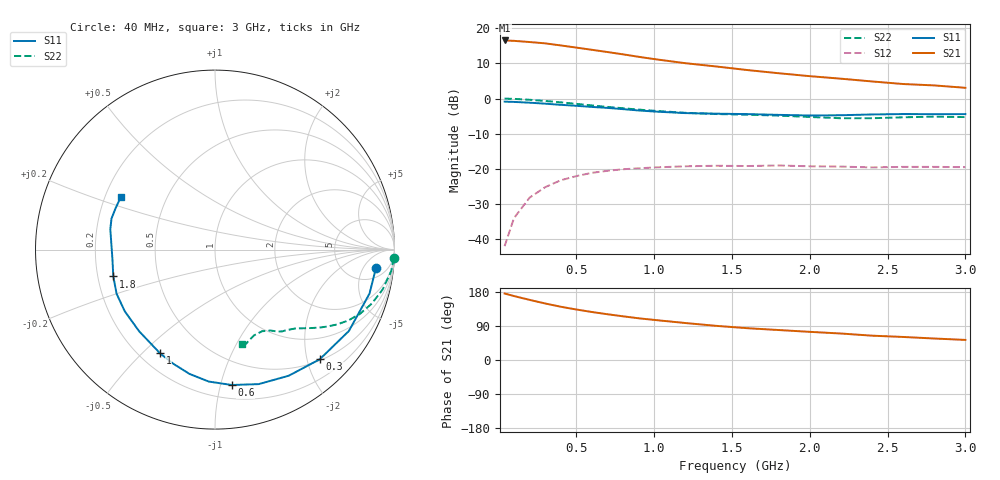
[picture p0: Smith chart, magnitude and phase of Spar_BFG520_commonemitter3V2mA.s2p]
! Filename:  BFG520A.S2P  Version:  2.1
! NXP part #: BFG520  Date: Feb 1992
! Bias condition: Vce=3V, Ic=2mA
! IN LINE PINNING: same data as with cross emitter pinning.
#  MHz  S  MA  R  50
! Freq  S11  S21  S12  S22  !GUM [dB]
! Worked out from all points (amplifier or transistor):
!   21 points, 40 MHz to 3 GHz, reference 50 ohm
!   highest |S21| = 16.5 dB at 40 MHz (marker M1)
!   |S21| within 3 dB of that: start of sweep to 655.1 MHz
!   unconditionally stable (mu >= 1): 2.252 GHz to end of sweep
!   at 300 MHz: K = 0.09, MSG = 20.4 dB, |S12| = -25.2 dB
!   at 1 GHz: K = 0.38, MSG = 15.4 dB, |S12| = -19.6 dB
!   at 3 GHz: K = 1.25, MAG = 8.3 dB, |S12| = -19.5 dB
!   S11 on the Smith chart (normalised r, x): 40 MHz: 9, -10; 300 MHz: 0.52, -2.24; 600 MHz: 0.30, -1.08; 1 GHz: 0.28, -0.57; 1.8 GHz: 0.27, -0.12; 3 GHz: 0.27, +0.25
40  0.903 -6.4  6.678 175.4  0.008 85.5  0.997 -2.7
100  0.895 -15.9  6.594 168.8  0.02 81.6  0.989 -7.0
200  0.873 -31.3  6.344 158.7  0.039 72.5  0.96 -13.4
300  0.845 -46.3  6.077 149.2  0.055 65.5  0.924 -19.0
400  0.814 -59.7  5.679 140.6  0.069 59.1  0.883 -24.0
500  0.788 -72.0  5.29 133.3  0.079 53.5  0.84 -28.1
600  0.76 -83.0  4.922 126.7  0.088 48.5  0.798 -31.5
700  0.736 -92.7  4.575 120.8  0.094 44.5  0.76 -34.3
800  0.707 -101.6  4.242 115.3  0.099 41.4  0.728 -36.6
900  0.677 -110.1  3.916 110.1  0.102 38.5  0.697 -38.8
1000  0.654 -117.9  3.633 105.8  0.105 36.3  0.67 -40.8
1200  0.621 -132.9  3.176 97.6  0.109 32.8  0.627 -44.5
1400  0.609 -145.6  2.85 90.1  0.111 29.6  0.602 -48.1
1600  0.601 -155.8  2.536 83.9  0.11 29.1  0.589 -50.7
1800  0.586 -165.2  2.287 79.1  0.112 28.5  0.572 -52.9
2000  0.574 -174.6  2.078 74.3  0.109 28.4  0.547 -55.5
2200  0.579 176.3  1.913 69.9  0.108 28.2  0.525 -60.0
2400  0.594 169.1  1.748 64.2  0.105 29.7  0.525 -65.5
2600  0.602 163.4  1.607 60.8  0.107 31.9  0.541 -69.7
2800  0.6 157.6  1.535 56.7  0.107 32.9  0.553 -71.8
3000  0.601 150.6  1.42 53.0  0.106 36.2  0.545 -73.9
